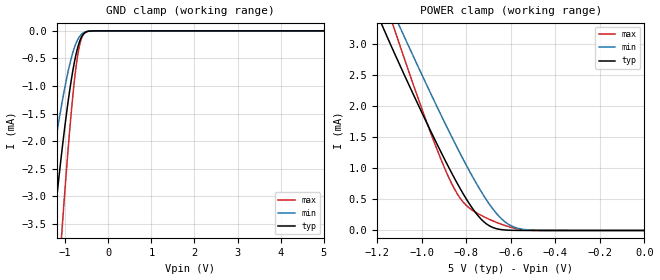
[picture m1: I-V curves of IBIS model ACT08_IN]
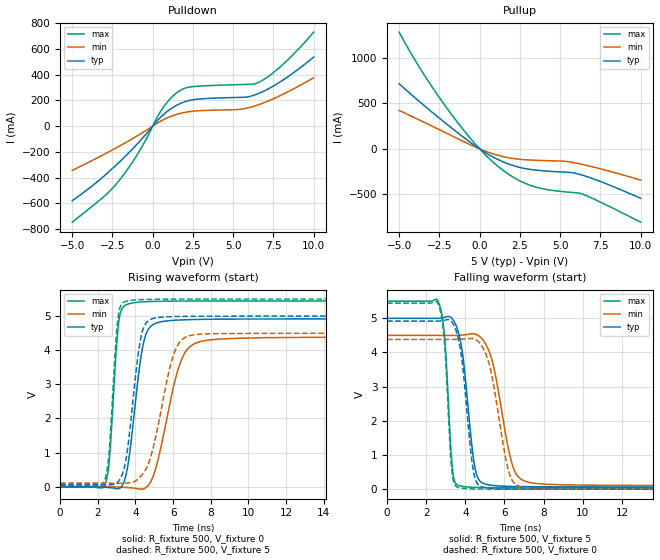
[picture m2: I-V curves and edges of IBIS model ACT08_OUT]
| TEXAS INSTRUMENTS INCORPORATED
| Standard Linear and Logic Group
| IBIS Model of SN74ACT08
| QUADRUPLE 2-INPUT POSITIVE-AND GATES
| This file contains package information for the following:
|  SOIC 14-pin (D) package as [Component] ACT08_D
|  SSOP 14-pin (DB) package as [Component] ACT08_DB
|  PDIP 14-pin (N) package as [Component] ACT08_N
|  SOP 14-pin (NS) package as [Component] ACT08_NS
|  TSSOP 14-pin (PW) package as [Component] ACT08_PW
| This device can be powered at the following Vccs:
|  5 volt Vcc
| This file provides unique models under the [Model Selector] for each Vcc.
| For operation at a specific Vcc, select the appropriate model after each
| [Model Selector] keyword.
[IBIS Ver]   3.2
[Comment char]  |_char
[File Name]   sn74act08.ibs
[File Rev]   1.1 | x_die
[Date]   February 19, 2003
[Source]   Data created from TI-SPICE simulations at TI-SLL.
[Notes]   The following is an IBIS list for the ACT08.
   Please contact sllibis@ti.com with questions and
   comments concerning SLL IBIS models.
   This IBIS model is created from a BA (back annotated
   netlist)
   - C_comp values are taken at a different test condition than
   the Ci in data sheet.
[Disclaimer] Property of Texas Instruments Incorporated.  Unauthorized
   reproduction and/or distribution is strictly prohibited.
   This product is protected under copyright law.
   Created  2003, (C) Copyright  2003, Texas Instruments
   Incorporated, All Rights Reserved
   UNLESS THERE IS A SIGNED, WRITTEN AGREEMENT TO THE
   CONTRARY, TEXAS INSTRUMENTS (TI) IS PROVIDING THE IBIS
   MODELS  AND WITHOUT ANY WARRANTY, EXPRESSED OR
   IMPLIED.  TI assumes no liability for:
   1) the accuracy of the IBIS models provided to your
   company;
   2) the proper functioning of these IBIS Models in your
   design or for any resulting applications; or
   3) infringement of patents, copyrights or intellectual
   property rights resulting from your use of these IBIS
   models.
   TI provides IBIS Models as a service to our customers.
   You and your company shall not distribute, sell or give
   these models to anyone else without prior written
   permission from TI.
   TI reserves the right to make changes to our products or
   to discontinue any semiconductor product or service
   without notice, and advises our customers to obtain the
   latest version of relevant information to verify, before
   placing orders, that the information being relied on is
   current.
   Please be aware that your receipt and use of the IBIS
   information provided shall serve as acceptance of these
   terms and conditions.  If you do not accept these terms,
   you should return or destroy the IBIS models and any
   other accompanying information immediately.
| Component ACT08_D 14-pin SOIC
[Component]   ACT08_D
[Manufacturer]   Texas Instruments, Inc.
[Package]
|   typ   min   max
R_pkg   3.100e-02   2.800e-02   3.400e-02
L_pkg   3.109e-09   2.462e-09   3.889e-09
C_pkg   4.730e-13   3.630e-13   6.280e-13
[Pin]   signal_name   model_name   R_pin   L_pin   C_pin
1   1A   ACT08_IN   3.300e-02   3.854e-09   6.220e-13
2   1B   ACT08_IN   3.200e-02   3.188e-09   4.730e-13
3   1Y   ACT08_OUT   2.800e-02   2.462e-09   3.770e-13
4   2A   ACT08_IN   3.100e-02   2.596e-09   3.630e-13
5   2B   ACT08_IN   2.800e-02   2.521e-09   3.720e-13
6   2Y   ACT08_OUT   3.400e-02   3.250e-09   4.760e-13
7   GND   GND   3.400e-02   3.889e-09   6.280e-13
8   3Y   ACT08_OUT   3.400e-02   3.889e-09   6.280e-13
9   3A   ACT08_IN   3.400e-02   3.250e-09   4.760e-13
10   3B   ACT08_IN   2.800e-02   2.521e-09   3.720e-13
11   4Y   ACT08_OUT   3.100e-02   2.596e-09   3.640e-13
12   4A   ACT08_IN   2.800e-02   2.462e-09   3.770e-13
13   4B   ACT08_IN   3.200e-02   3.188e-09   4.730e-13
14   VCC   POWER   3.300e-02   3.854e-09   6.220e-13
| Component ACT08_DB 14-pin SSOP
[Component]   ACT08_DB
[Manufacturer]   Texas Instruments, Inc.
[Package]
|   typ   min   max
R_pkg   4.400e-02   4.100e-02   4.600e-02
L_pkg   3.551e-09   3.258e-09   3.927e-09
C_pkg   4.020e-13   3.600e-13   4.210e-13
[Pin]   signal_name   model_name   R_pin   L_pin   C_pin
1   1A   ACT08_IN   4.600e-02   3.927e-09   4.080e-13
2   1B   ACT08_IN   4.400e-02   3.587e-09   4.210e-13
3   1Y   ACT08_OUT   4.100e-02   3.289e-09   3.980e-13
4   2A   ACT08_IN   4.200e-02   3.258e-09   3.600e-13
5   2B   ACT08_IN   4.100e-02   3.286e-09   4.030e-13
6   2Y   ACT08_OUT   4.400e-02   3.586e-09   4.210e-13
7   GND   GND   4.600e-02   3.927e-09   4.080e-13
8   3Y   ACT08_OUT   4.600e-02   3.927e-09   4.080e-13
9   3A   ACT08_IN   4.400e-02   3.586e-09   4.210e-13
10   3B   ACT08_IN   4.100e-02   3.286e-09   4.030e-13
11   4Y   ACT08_OUT   4.300e-02   3.258e-09   3.600e-13
12   4A   ACT08_IN   4.100e-02   3.289e-09   3.980e-13
13   4B   ACT08_IN   4.400e-02   3.587e-09   4.210e-13
14   VCC   POWER   4.600e-02   3.927e-09   4.080e-13
| Component ACT08_N 14-pin PDIP
[Component]   ACT08_N
[Manufacturer]   Texas Instruments, Inc.
[Package]
|   typ   min   max
R_pkg   4.500e-02   3.700e-02   6.300e-02
L_pkg   5.407e-09   3.922e-09   6.942e-09
C_pkg   3.890e-13   2.050e-13   6.040e-13
[Pin]   signal_name   model_name   R_pin   L_pin   C_pin
1   1A   ACT08_IN   6.300e-02   6.942e-09   6.040e-13
2   1B   ACT08_IN   3.700e-02   6.200e-09   4.060e-13
3   1Y   ACT08_OUT   4.200e-02   4.389e-09   3.220e-13
4   2A   ACT08_IN   3.800e-02   3.922e-09   2.050e-13
5   2B   ACT08_IN   3.900e-02   4.301e-09   2.980e-13
6   2Y   ACT08_OUT   3.800e-02   5.329e-09   3.560e-13
7   GND   GND   5.300e-02   6.510e-09   5.440e-13
8   3Y   ACT08_OUT   5.300e-02   6.437e-09   5.390e-13
9   3A   ACT08_IN   3.900e-02   5.352e-09   3.470e-13
10   3B   ACT08_IN   4.200e-02   4.473e-09   2.970e-13
11   4Y   ACT08_OUT   4.400e-02   4.326e-09   2.250e-13
12   4A   ACT08_IN   4.200e-02   4.295e-09   2.800e-13
13   4B   ACT08_IN   4.200e-02   6.318e-09   4.180e-13
14   VCC   POWER   6.100e-02   6.900e-09   6.030e-13
| Component ACT08_NS 14-pin SOP
[Component]   ACT08_NS
[Manufacturer]   Texas Instruments, Inc.
[Package]
|   typ   min   max
R_pkg   4.500e-02   3.900e-02   5.400e-02
L_pkg   3.796e-09   2.561e-09   4.952e-09
C_pkg   5.280e-13   2.880e-13   7.100e-13
[Pin]   signal_name   model_name   R_pin   L_pin   C_pin
1   1A   ACT08_IN   4.700e-02   4.867e-09   7.060e-13
2   1B   ACT08_IN   5.100e-02   4.083e-09   5.920e-13
3   1Y   ACT08_OUT   4.100e-02   2.915e-09   3.760e-13
4   2A   ACT08_IN   3.900e-02   2.561e-09   2.880e-13
5   2B   ACT08_IN   4.100e-02   3.101e-09   4.300e-13
6   2Y   ACT08_OUT   4.700e-02   4.047e-09   5.890e-13
7   GND   GND   5.100e-02   4.909e-09   7.000e-13
8   3Y   ACT08_OUT   4.500e-02   4.784e-09   6.940e-13
9   3A   ACT08_IN   5.400e-02   4.176e-09   5.970e-13
10   3B   ACT08_IN   3.900e-02   3.287e-09   4.490e-13
11   4Y   ACT08_OUT   3.900e-02   2.586e-09   2.940e-13
12   4A   ACT08_IN   4.000e-02   2.802e-09   3.710e-13
13   4B   ACT08_IN   4.900e-02   4.080e-09   5.930e-13
14   VCC   POWER   5.200e-02   4.952e-09   7.100e-13
| Component ACT08_PW 14-pin TSSOP
[Component]   ACT08_PW
[Manufacturer]   Texas Instruments, Inc.
[Package]
|   typ   min   max
R_pkg   3.200e-02   2.900e-02   3.500e-02
L_pkg   2.378e-09   2.170e-09   2.680e-09
C_pkg   3.140e-13   2.700e-13   3.350e-13
[Pin]   signal_name   model_name   R_pin   L_pin   C_pin
1   1A   ACT08_IN   3.300e-02   2.618e-09   3.300e-13
2   1B   ACT08_IN   3.100e-02   2.313e-09   3.170e-13
3   1Y   ACT08_OUT   3.000e-02   2.310e-09   3.140e-13
4   2A   ACT08_IN   3.100e-02   2.173e-09   2.720e-13
5   2B   ACT08_IN   3.000e-02   2.204e-09   3.090e-13
6   2Y   ACT08_OUT   3.200e-02   2.315e-09   3.170e-13
7   GND   GND   3.500e-02   2.680e-09   3.350e-13
8   3Y   ACT08_OUT   3.300e-02   2.640e-09   3.330e-13
9   3A   ACT08_IN   3.400e-02   2.347e-09   3.190e-13
10   3B   ACT08_IN   2.900e-02   2.277e-09   3.130e-13
11   4Y   ACT08_OUT   3.100e-02   2.170e-09   2.700e-13
12   4A   ACT08_IN   3.100e-02   2.244e-09   3.110e-13
13   4B   ACT08_IN   3.300e-02   2.343e-09   3.210e-13
14   VCC   POWER   3.500e-02   2.657e-09   3.320e-13
| Models and submodels in the file (2): ACT08_IN (Input), ACT08_OUT (Output)
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[Model]   ACT08_IN
Model_type  Input
Vinl = 0.8
Vinh = 2.0
| variable   typ   min   max
C_comp   4.5pF   NA   NA
[Temperature Range]   40   100   -40
| Ambient temperature   25   85   -40
[Voltage range]   5   4.5   5.5
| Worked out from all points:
|   GND clamp passes 1 mA (typ) near -0.88 V on its own axis
|   POWER clamp passes 1 mA (typ) near -0.88 V on its own axis
[GND Clamp]
| ACT08_IN
|   Voltage   I(typ)   I(min)   I(max)
-5V       -46.92mA   -30.58mA   -59.62mA
-1.56V    -6.035mA   -3.826mA   -9.528mA
-1.51V    -5.59mA    -3.537mA   -8.882mA
-1.305V   -3.869mA   -2.418mA   -6.312mA
-1.255V   -3.478mA   -2.163mA   -5.708mA
-1.08V    -2.21mA    -1.334mA   -3.692mA
-1.06V    -2.076mA   -1.247mA   -3.474mA
-900mV    -1.111mA   -628.4uA   -1.852mA
-770mV    -508.4uA   -270.1uA   -799.3uA
-670mV    -203.9uA   -108.8uA   -280.1uA
-550mV    -38.99uA   -24.34uA   -40.29uA
5V        16.38nA    4.859uA    150.6nA
[POWER Clamp]
| ACT08_IN
|   Voltage   I(typ)   I(min)   I(max)
-5V       45.74mA    45.24mA    49.64mA
-1.17V    3.235mA    3.838mA    3.746mA
-1.125V   2.87mA     3.482mA    3.262mA
-1.075V   2.477mA    3.09mA     2.732mA
-965mV    1.638mA    2.244mA    1.62mA
-895mV    1.129mA    1.722mA    985.3uA
-840mV    755.6uA    1.327mA    587.5uA
-785mV    423.6uA    951.8uA    357.6uA
-695mV    72.53uA    417uA      176.8uA
-640mV    12.79uA    181.6uA    97.2uA
-585mV    1.851uA    53.91uA    37.94uA
-84.45fV  16.38nA    947.5pA    229.7nA
[Model]   ACT08_OUT
Model_type  Output
Vref =   0
Rref =   500
Cref =   50p
Vmeas =   1.5
| variable   typ   min   max
C_comp   13.36pF   5.61pF   24.96pF
| C_pullup   14.74pF   5.61pF   24.96pF
| C_pulldown   11.98pF   5.98pF   19.94pF
[Temperature Range]   40   100   -40
| Ambient temperature   25   85   -40
[Voltage range]   5   4.5   5.5
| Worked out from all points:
|   slope of the pulldown table from 0 to 0.75 V, typ, clamps not added: 7.64 ohm
|   slope of the pullup table from 0 to 0.75 V, typ, clamps not added: 9.15 ohm
|   rising waveform, R_fixture 500, V_fixture 0: 20-80 % time 639ps typ, 1.07ns min, 373ps max; typ from 0 V to 4.92 V
|   falling waveform, R_fixture 500, V_fixture 5: 20-80 % time 534ps typ, 846ps min, 319ps max; typ from 5 V to 0.063 V
|   rising waveform, R_fixture 500, V_fixture 5: 20-80 % time 614ps typ, 1.02ns min, 364ps max; typ from 0.063 V to 5 V
|   falling waveform, R_fixture 500, V_fixture 0: 20-80 % time 511ps typ, 785ps min, 309ps max; typ from 4.92 V to 0 V
[Pulldown]
| ACT08_OUT
|   Voltage   I(typ)   I(min)   I(max)
-5V       -580.4mA   -344.3mA   -746.8mA
-3V       -385.5mA   -218.2mA   -544mA
-2.135V   -286.7mA   -160.2mA   -430.5mA
-865mV    -125.8mA   -68.55mA   -201.6mA
555mV     76.37mA    42.29mA    127mA
1.47V     159.9mA    89.76mA    256.7mA
1.91V     184.9mA    104mA      290.3mA
2.405V    202.4mA    114.2mA    305.1mA
5.375V    222.9mA    129.7mA    322mA
6.535V    250.9mA    164.4mA    337.7mA
8.04V     353.5mA    244.3mA    473.4mA
10V       536.5mA    375.2mA    730.1mA
[Pullup]
| ACT08_OUT
|   Voltage   I(typ)   I(min)   I(max)
-5V       714.7mA    422.3mA    1.282A
-3.495V   482.8mA    295.7mA    826.6mA
-1.81V    239.1mA    150.5mA    393.9mA
-145mV    17.72mA    11.1mA     28.11mA
570mV     -63.95mA   -39.32mA   -102.7mA
1.285V    -129.4mA   -77.34mA   -212.7mA
2.305V    -195.1mA   -111mA     -333.4mA
3.33V     -230.3mA   -124.6mA   -411.9mA
5.235V    -255.6mA   -135.9mA   -471.4mA
6.175V    -279mA     -163.2mA   -486.7mA
7.215V    -339.4mA   -206.5mA   -560.8mA
10V       -543.6mA   -343.1mA   -805.8mA
[Ramp]
| ACT08_OUT
| variable   typ   min   max
dV/dt_r   2.99/6.49E-10   2.67/1.09E-09   3.29/3.79E-10
dV/dt_f   3.00/5.47E-10   2.67/8.61E-10   3.31/3.29E-10
R_load = 500
[Rising Waveform]
| ACT08_OUT
R_fixture =   500
C_fixture =   0
L_fixture =   0
V_fixture =   0
V_fixture_min = 0
V_fixture_max = 0
|   Time   V(typ)   V(min)   V(max)
0s        1.229nV    2.108nV    789.1pV
2.39ns    -17.48mV   260.9uV    70.27mV
2.62ns    -27.99mV   -1.862mV   842.6mV
3.135ns   -52.62mV   -13.03mV   4.911V
3.805ns   1.504V     -37.01mV   5.383V
4.29ns    3.8V       -72.57mV   5.414V
4.68ns    4.611V     40.52mV    5.425V
6.43ns    4.888V     3.703V     5.441V
7.685ns   4.906V     4.282V     5.442V
50ns      4.918V     4.383V     5.443V
[Falling Waveform]
| ACT08_OUT
R_fixture =   500
C_fixture =   0
L_fixture =   0
V_fixture =   5
V_fixture_min = 4.5
V_fixture_max = 5.5
|   Time   V(typ)   V(min)   V(max)
0s        5V         4.5V       5.5V
2.645ns   5V         4.5V       5.447V
2.94ns    5.029V     4.5V       4.453V
3.35ns    4.976V     4.499V     544.3mV
3.71ns    4.434V     4.505V     95.82mV
4.505ns   590.2mV    4.538V     52.97mV
5.265ns   119.5mV    3.955V     46.07mV
6.43ns    79.55mV    660.3mV    42.74mV
7.465ns   72.18mV    176.2mV    41.65mV
50ns      63.36mV    104.1mV    40.77mV
[Rising Waveform]
| ACT08_OUT
R_fixture =   500
C_fixture =   0
L_fixture =   0
V_fixture =   5
V_fixture_min = 4.5
V_fixture_max = 5.5
|   Time   V(typ)   V(min)   V(max)
0s        63.36mV    104.1mV    40.77mV
2.35ns    53mV       104.3mV    163.5mV
2.595ns   53.65mV    102.6mV    978.8mV
3.085ns   145.5mV    98.07mV    4.997V
3.645ns   1.395V     111.9mV    5.452V
4.145ns   3.888V     226.9mV    5.481V
4.49ns    4.731V     455mV      5.488V
6.045ns   4.987V     3.9V       5.498V
7.06ns    4.993V     4.449V     5.5V
50ns      5V         4.5V       5.5V
[Falling Waveform]
| ACT08_OUT
R_fixture =   500
C_fixture =   0
L_fixture =   0
V_fixture =   0
V_fixture_min = 0
V_fixture_max = 0
|   Time   V(typ)   V(min)   V(max)
0s        4.918V     4.383V     5.443V
2.615ns   4.918V     4.383V     5.414V
2.935ns   4.944V     4.382V     4.298V
3.32ns    4.885V     4.382V     500.3mV
3.695ns   4.256V     4.387V     39.37mV
4.42ns    507mV      4.404V     7.378mV
5.07ns    37.57mV    3.917V     2.827mV
6.23ns    4.689mV    489.5mV    878.2uV
7.065ns   2.244mV    41.61mV    440.5uV
50ns      -3.202nV   -6.29nV    -4.249nV
